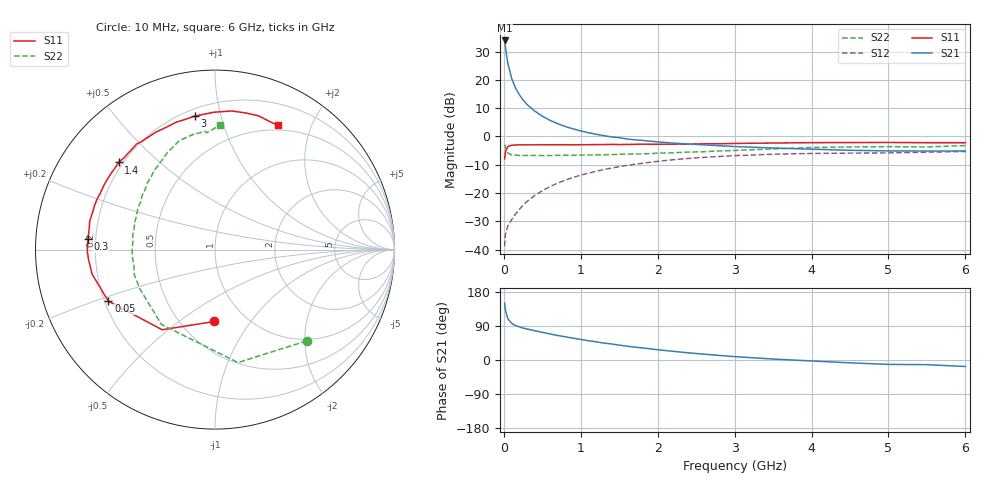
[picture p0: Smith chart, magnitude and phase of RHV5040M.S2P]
! SIEMENS Small Signal Semiconductors
! BFR106
! Si NPN RF Bipolar Junction Transistor in SOT23
! VCE = 0.5 V  IC = 40 mA
! Common Emitter S-Parameters:  August  1996
# GHz  S  MA  R  50
!  f  S11  S21  S12  S22
! GHz  MAG  ANG  MAG  ANG  MAG  ANG  MAG  ANG
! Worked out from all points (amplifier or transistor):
!   36 points, 10 MHz to 6 GHz, reference 50 ohm
!   highest |S21| = 33.9 dB at 10 MHz (marker M1)
!   |S21| within 3 dB of that: start of sweep to 24.03 MHz
!   unconditionally stable (mu >= 1): 163.1 MHz to end of sweep
!   at 250 MHz: K = 1.12, MAG = 16.5 dB, |S12| = -24.3 dB
!   at 1.4 GHz: K = 1.14, MAG = 3.2 dB, |S12| = -11.2 dB
!   at 6 GHz: K = 1.03, MAG = -1.0 dB, |S12| = -5.3 dB
!   S11 on the Smith chart (normalised r, x): 10 MHz: 0.72, -0.69; 50 MHz: 0.22, -0.22; 300 MHz: 0.17, +0.04; 1.4 GHz: 0.18, +0.37; 3 GHz: 0.24, +0.83; 6 GHz: 0.44, +1.53
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0.01  0.4004 -90.4  49.82 150.2  0.0115 65.6  0.7208 -44.9
0.02  0.535 -123.4  38.45 131.9  0.0183 52.3  0.6422 -78.5
0.05  0.6601 -154.2  20.21 109.3  0.0259 43.3  0.5126 -125.6
0.1  0.6986 -168.8  10.82 97.1  0.0337 48.8  0.4724 -152.4
0.15  0.7066 -175.6  7.291 91.3  0.0421 55.0  0.4711 -162.8
0.2  0.7118 -179.3  5.537 87.4  0.0512 59.0  0.4604 -168.7
0.25  0.7098 177.6  4.414 84.3  0.0608 62.0  0.4611 -173.1
0.3  0.7105 175.2  3.696 81.9  0.0706 64.0  0.4623 -175.7
0.4  0.7103 170.6  2.819 77.3  0.0902 65.2  0.4618 179.8
0.5  0.7161 167.1  2.288 73.1  0.1097 65.4  0.4602 176.2
0.6  0.7128 163.1  1.927 68.7  0.1301 64.7  0.46 173.6
0.7  0.7145 159.7  1.682 64.6  0.1497 63.6  0.4642 171.1
0.8  0.7146 156.9  1.497 61.2  0.1691 62.2  0.4655 168.4
1.1  0.7168 146.5  1.167 50.8  0.225 57.4  0.4716 161.9
1.4  0.7241 137.9  0.982 42.3  0.2763 51.6  0.479 155.4
1.7  0.7261 129.3  0.874 33.9  0.3222 45.9  0.4907 149.2
2.2  0.7325 116.7  0.764 22.9  0.3875 36.3  0.514 139.2
3  0.7523 98.7  0.664 8.9  0.4582 22.0  0.5657 124.1
3.5  0.7656 90.4  0.626 2.5  0.4856 14.4  0.6028 116.0
4.5  0.7805 77.2  0.57 -7.5  0.5075 1.3  0.6528 101.0
5.5  0.776 67.0  0.553 -12.3  0.5281 -6.3  0.6525 94.0
6  0.7751 63.3  0.554 -17.1  0.5417 -12.2  0.692 87.9
